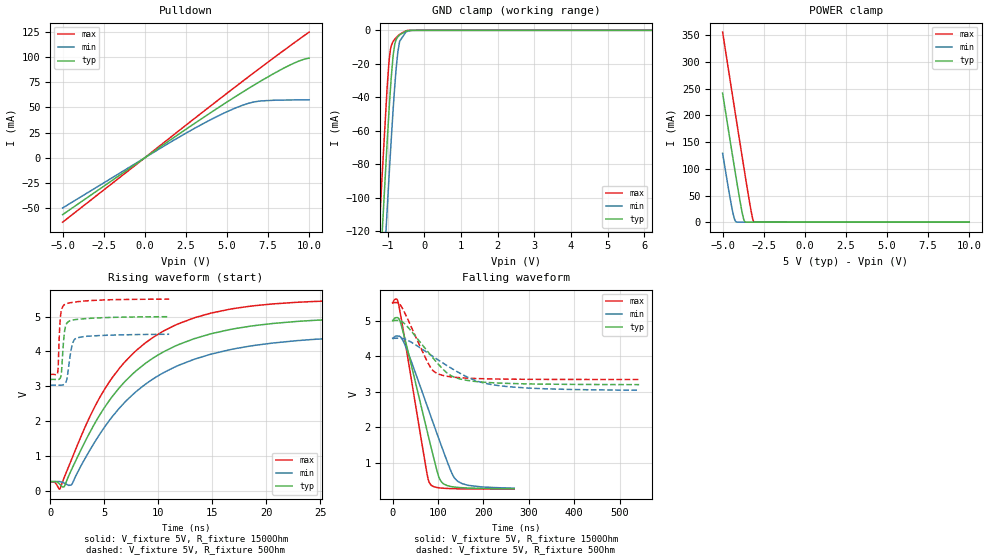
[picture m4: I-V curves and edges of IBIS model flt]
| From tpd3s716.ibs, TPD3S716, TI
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|   flt Model
[Model]   flt
Model_type   I/O_open_drain
Polarity   Non-Inverting
Vinl = 0.8
Vinh = 1.2
Vmeas = 2.5
Vref = 5
Cref = 2pF
Rref = 1500
|   typ   min   max
|   (nom PVT)   (fast PVT)   (slow PVT)
C_comp   5.357e-13   5.249e-13   5.856e-13
| Where nom  PVT is Nominal Process, 5V, 40C
|   Fast PVT is Strong Process,  5.5V, -40C
|   Slow PVT is Weak Process,   4.5V, 125C
[Voltage Range]   5   4.5   5.5
|Junction Temperature
[Temperature Range]   40   125   -40
[Pullup Reference]   5   4.5   5.5
[Pulldown Reference]   0   0   0
[Power Clamp Reference]   5   4.5   5.5
[GND Clamp Reference]   0   0   0
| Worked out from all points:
|   slope of the pulldown table from 0 to 0.75 V, typ, clamps not added: 86.9 ohm
|   GND clamp passes 1 mA (typ) near -0.54 V on its own axis
|   POWER clamp passes 1 mA (typ) near -3.64 V on its own axis
|   falling waveform, V_fixture 5V, R_fixture 1500Ohm: 20-80 % time 53.6ns typ, 70.8ns min, 40.7ns max; typ from 5 V to 0.282 V
|   rising waveform, V_fixture 5V, R_fixture 1500Ohm: 20-80 % time 8.01ns typ, 8.75ns min, 7.28ns max; typ from 0.275 V to 5 V
|   falling waveform, V_fixture 5V, R_fixture 50Ohm: 20-80 % time 71.8ns typ, 115ns min, 47.1ns max; typ from 5 V to 3.2 V
|   rising waveform, V_fixture 5V, R_fixture 50Ohm: 20-80 % time 283ps typ, 442ps min, 214ps max; typ from 3.2 V to 5 V
[Pulldown]
|   Voltage   I(typ)   I(min)   I(max)
-5V       -56.41mA   -49.77mA   -63.88mA
1.899V    21.62mA    18.77mA    24.64mA
3.744V    41.99mA    35.61mA    48.24mA
5.247V    58mA       47.59mA    67.2mA
6.322V    69.02mA    54.21mA    80.6mA
6.97V     75.41mA    56.31mA    88.59mA
8.935V    92.95mA    57.45mA    112.4mA
9.68V     97.83mA    57.55mA    121.1mA
10V       99.03mA    57.58mA    124.8mA
[GND Clamp]
|   Voltage   I(typ)   I(min)   I(max)
-5V       -1.862A    -1.873A    -1.865A
-1.225V   -152.8mA   -193.5mA   -118.4mA
-1.157V   -124.4mA   -165.4mA   -89.81mA
-1.012V   -66.87mA   -107.4mA   -34.04mA
-963mV    -48.7mA    -88.32mA   -19.23mA
-924.5mV  -35.64mA   -73.93mA   -11.78mA
-842mV    -13.8mA    -45.06mA   -6.434mA
-805mV    -8.404mA   -33.49mA   -5.324mA
-755mV    -5.02mA    -20.11mA   -4.096mA
-671mV    -2.758mA   -6.511mA   -2.391mA
-500mV    -522uA     -983.2uA   -256.6uA
10V       0A         0A         0A
[POWER Clamp]
|   Voltage   I(typ)   I(min)   I(max)
-5V       241.8mA    129.1mA    356.3mA
-4.438V   132.6mA    27.27mA    245.3mA
-4.303V   106.8mA    8.374mA    218.8mA
-4.248V   96.5mA     3.52mA     208.2mA
-4.16V    79.82mA    420.1uA    190.8mA
-3.875V   28.4mA     122.8nA    135.2mA
-3.695V   3.579mA    12.21nA    100.4mA
-3.62V    400.4uA    11.25nA    86.03mA
-3.272V   0A         0A         21.92mA
-3.163V   0A         0A         5.604mA
-3.091V   0A         0A         559.8uA
10V       0A         0A         0A
[Ramp]
R_load = 1500
|   typ   min   max
dV/dt_r   2.83519/8.00652e-09   2.53278/8.73001e-09   3.13904/7.28253e-09
dV/dt_f   2.8341/5.36473e-08   2.52913/7.09736e-08   3.13877/4.06087e-08
[Falling Waveform]
V_fixture = 5V
V_fixture_min = 4.5V
V_fixture_max = 5.5V
R_fixture = 1500Ohm
|   Time   V(typ)   V(min)   V(max)
0s        5V         4.5V       5.5V
8.488ns   5.083V     4.565V     5.602V
13.29ns   5.061V     4.564V     5.453V
32.33ns   4.217V     4.156V     4.043V
75.07ns   1.952V     2.641V     757.7mV
81.08ns   1.637V     2.425V     449.5mV
106.3ns   495.8mV    1.527V     302.2mV
130ns     341.3mV    732.2mV    285.5mV
141.4ns   322.5mV    512.7mV    281.7mV
267.6ns   281.6mV    299.7mV    270.4mV
[Rising Waveform]
V_fixture = 5V
V_fixture_min = 4.5V
V_fixture_max = 5.5V
R_fixture = 1500Ohm
|   Time   V(typ)   V(min)   V(max)
0s        274.7mV    278.6mV    268.3mV
877.2ps   202.9mV    276.8mV    59.15mV
1.266ns   122.9mV    237.4mV    373.2mV
1.935ns   595.7mV    177.2mV    881mV
4.411ns   2.094V     1.55V      2.586V
6.987ns   3.161V     2.571V     3.726V
10.45ns   3.98V      3.383V     4.576V
14.78ns   4.497V     3.913V     5.088V
27.14ns   4.928V     4.393V     5.457V
60.22ns   4.999V     4.498V     5.5V
[Falling Waveform]
V_fixture = 5V
V_fixture_min = 4.5V
V_fixture_max = 5.5V
R_fixture = 50Ohm
|   Time   V(typ)   V(min)   V(max)
0s        5V         4.5V       5.5V
16.26ns   4.997V     4.502V     5.453V
33.47ns   4.816V     4.444V     5.034V
79.29ns   4.098V     4.074V     3.778V
89.83ns   3.936V     3.983V     3.584V
102.5ns   3.75V      3.876V     3.492V
140.2ns   3.392V     3.58V      3.404V
179.7ns   3.295V     3.331V     3.375V
226.6ns   3.251V     3.187V     3.361V
543.2ns   3.202V     3.045V     3.346V
[Rising Waveform]
V_fixture = 5V
V_fixture_min = 4.5V
V_fixture_max = 5.5V
R_fixture = 50Ohm
|   Time   V(typ)   V(min)   V(max)
0s        3.2V       3.035V     3.345V
682.5ps   3.194V     3.035V     3.389V
720.7ps   3.195V     3.034V     3.502V
939.8ps   3.25V      3.032V     4.984V
1.029ns   3.38V      3.034V     5.17V
1.345ns   4.62V      3.078V     5.347V
1.569ns   4.822V     3.255V     5.376V
2.032ns   4.898V     4.191V     5.404V
2.453ns   4.917V     4.388V     5.422V
11.02ns   4.995V     4.493V     5.497V
